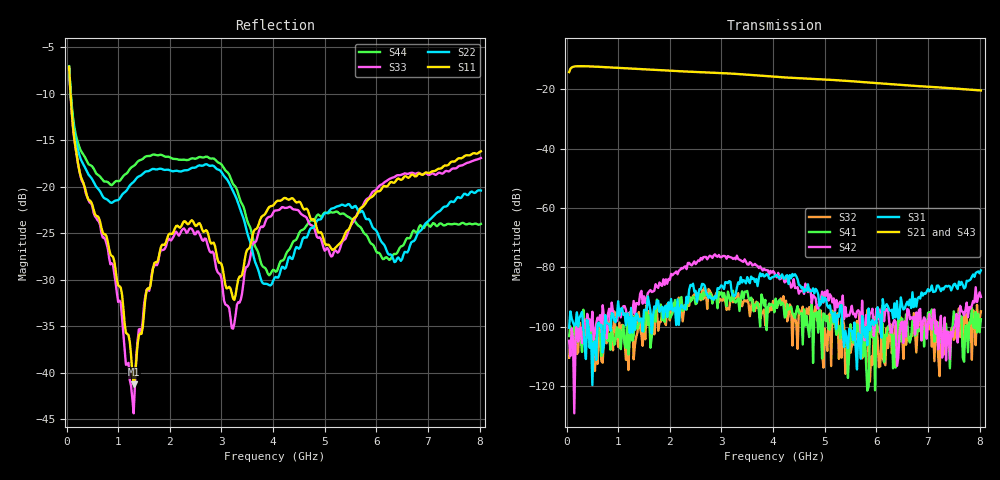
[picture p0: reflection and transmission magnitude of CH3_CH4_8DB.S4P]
!Agilent Technologies,E5071C,MY46316741,A.11.02
!Date: Thu May 28 15:02:58 2026
!Data & Calibration Information:
!1:CH3 INPUT 2:CH3 OUTPUT 3:CH4 INPUT 4:CH4 OUTPUT
!Freq	S11:SOLT4(ON)	S12:SOLT4(ON)	S13:SOLT4(ON)	S14:SOLT4(ON)
!	S21:SOLT4(ON)	S22:SOLT4(ON)	S23:SOLT4(ON)	S24:SOLT4(ON)
!	S31:SOLT4(ON)	S32:SOLT4(ON)	S33:SOLT4(ON)	S34:SOLT4(ON)
!	S41:SOLT4(ON)	S42:SOLT4(ON)	S43:SOLT4(ON)	S44:SOLT4(ON)
!PortZ  Port1:50+j0  Port2:50+j0  Port3:50+j0  Port4:50+j0
!Above PortZ is port z conversion or system Z0 setting when saving the data.
!When reading, reference impedance value at option line is always used.
# Hz S dB R 50
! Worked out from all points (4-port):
!   320 points, 50 MHz to 8.025 GHz, reference 50 ohm
!   strongest paths, dB at 50 MHz, 2.05 GHz, 4.05 GHz, 6.05 GHz, 8.025 GHz:
!     S21: -14.3, -13.9, -15.9, -18.0, -20.4
!     S43: -14.2, -13.9, -15.9, -18.1, -20.5
!     S31: -100.3, -94.6, -82.7, -96.7, -81.0
!     S42: -104.7, -82.7, -82.9, -94.1, -89.9
!     S41: -103.1, -95.6, -90.5, -101.7, -97.5
!     S32: -110.4, -92.5, -93.1, -113.6, -94.8
!   lowest |S11| = -41.3 dB at 1.3 GHz (marker M1), VSWR 1.02, Z = 49.2 - j0.37 ohm
!   |S11| at or under -10 dB: 78.3 MHz to end of sweep
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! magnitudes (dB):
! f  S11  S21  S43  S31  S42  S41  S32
! 50 MHz  -7.1  -14.3  -14.2  -100.3  -104.7  -103.1  -110.4
! 425 MHz  -21.4  -12.3  -12.3  -100.2  -97.9  -97.2  -100.8
! 1.3 GHz  -41.3  -13.2  -13.2  -96.9  -91.3  -103.1  -111.0
! 2.125 GHz  -24.2  -13.9  -13.9  -99.4  -81.4  -93.1  -92.4
! 3.225 GHz  -32.0  -14.8  -14.8  -89.5  -77.2  -87.9  -91.8
! 3.95 GHz  -22.1  -15.7  -15.7  -83.9  -81.2  -92.9  -93.4
! 8.025 GHz  -16.2  -20.4  -20.5  -81.0  -89.9  -97.5  -94.8
